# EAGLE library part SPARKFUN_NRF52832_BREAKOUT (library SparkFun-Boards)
SparkFun nRF52832 Breakout SoC microcontroller with BLE, ANT, Nordic support, and 2.4Ghz multiprotocol radio SparkFun Products: SparkFun nRF52832 Breakout
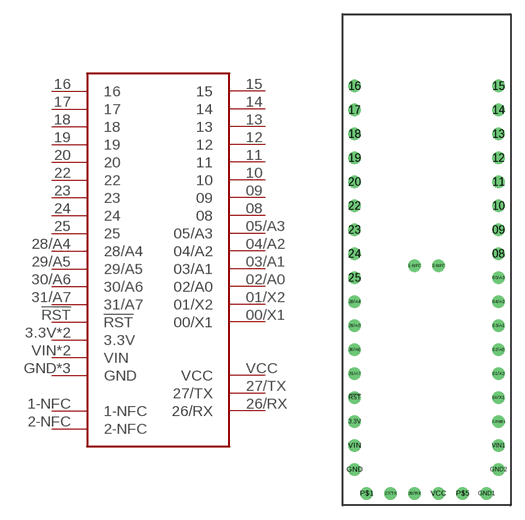
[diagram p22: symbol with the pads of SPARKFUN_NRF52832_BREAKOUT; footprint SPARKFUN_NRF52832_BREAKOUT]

Designator prefix B

## SPARKFUN_NRF52832_BREAKOUT (SF_ID: WRL-13990)  [SPARKFUN_NRF52832_BREAKOUT]
00/X1  00/X1
1-NFC  1-NFC
01/X2  01/X2
2-NFC  2-NFC
02/A0  02/A0
3.3V  3.3V
3.3V@1  3.3V
03/A1  03/A1
04/A2  04/A2
05/A3  05/A3
08  08
09  09
10  10
11  11
12  12
13  13
14  14
15  15
16  16
17  17
18  18
19  19
20  20
22  22
23  23
24  24
25  25
26/RX  26/RX
27/TX  27/TX
28/A4  28/A4
29/A5  29/A5
30/A6  30/A6
31/A7  31/A7
!RST  !RST
GND  GND
GND1  GND
GND2  GND
VCC  VCC
VIN  VIN
VIN1  VIN

## Footprint SPARKFUN_NRF52832_BREAKOUT (pad centres in mm)
SparkFun nRF42832 Breakout Specifications: Pin count:42 Pin pitch: 0.1" Area: 0.7x2.05 Example device(s): SPARKFUN_NRF42832_BREAKOUT
drill 0.8: 00/X1 16.51,11.43; 1-NFC 7.62,25.4; 01/X2 16.51,13.97; 2-NFC 10.16,25.4; 02/A0 16.51,16.51; 3.3V 1.27,8.89; 3.3V@1 16.51,8.89; 03/A1 16.51,19.05; 04/A2 16.51,21.59; 05/A3 16.51,24.13; 08 16.51,26.67; 09 16.51,29.21; 10 16.51,31.75; 11 16.51,34.29; 12 16.51,36.83; 13 16.51,39.37; 14 16.51,41.91; 15 16.51,44.45; 16 1.27,44.45; 17 1.27,41.91; 18 1.27,39.37; 19 1.27,36.83; 20 1.27,34.29; 22 1.27,31.75; 23 1.27,29.21; 24 1.27,26.67; 25 1.27,24.13; 26/RX 7.62,1.27; 27/TX 5.08,1.27; 28/A4 1.27,21.59; 29/A5 1.27,19.05; 30/A6 1.27,16.51; 31/A7 1.27,13.97; !RST 1.27,11.43; GND 1.27,3.81; GND1 15.24,1.27; GND2 16.51,3.81; P$1 2.54,1.27; P$5 12.7,1.27; VCC 10.16,1.27; VIN 1.27,6.35; VIN1 16.51,6.35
